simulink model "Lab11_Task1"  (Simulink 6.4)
settings: Solver=ode45  StartTime=0.0  StopTime=40  MaxStep=0.008  RelTol=1e-3
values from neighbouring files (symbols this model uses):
  B1 = 1/R1+D1    (= 5.99001338888)    [AGC_Data.m]
  D1 = 0.75/(2*pi*60)    (= 0.00198943678865)    [AGC_Data.m]
  DL1 = 1    [AGC_Data.m]
  DL2 = 0    [AGC_Data.m]
  K1 = 0.001*((2*pi*60))    (= 0.376991118431)    [AGC_Data.m]
  M1 = (2*H1)/(2*pi*60)    (= 0.0281173732796)    [AGC_Data.m]
  R1 = 0.167    [AGC_Data.m]
  T12 = 0.1    [AGC_Data.m]
  Tg1 = .26    (= 0.26)    [AGC_Data.m]
  thetar = 0    [AGC_Data.m]
  Ts1 = .26    (= 0.26)    [AGC_Data.m]

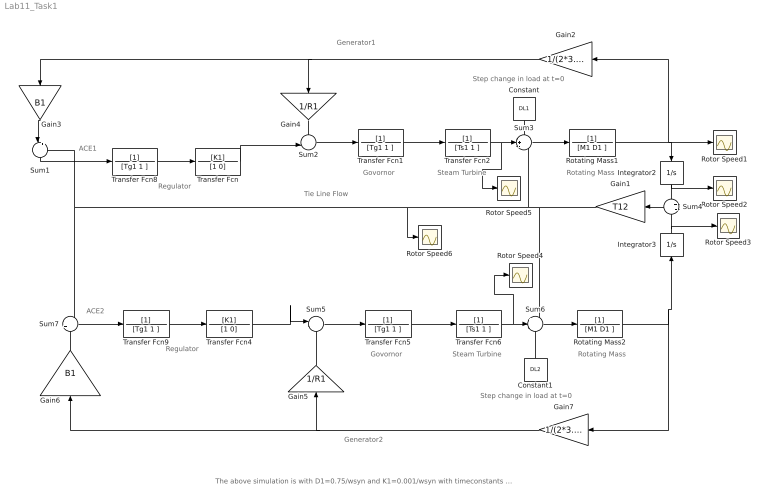
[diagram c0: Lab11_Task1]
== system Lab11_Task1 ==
  note: The above simulation is with D1=0.75/wsyn and K1=0.001/wsyn with timeconstants Tg1,Ts1 in seconds
  note: Generator1
  note: Generator2
  note: Rotating Mass
  note: Rotating Mass
  note: Step change in load at t=0
  note: Step change in load at t=0
  note: Tie Line Flow
  note: Govornor
  note: Steam Turbine
  note: Regulator
  note: Regulator
  note: Govornor
  note: Steam Turbine
  note: ACE1
  note: ACE2
  Constant : Constant  Orientation=down  Value=DL1  OutDataType=sfix(16)  ConRadixGroup=Use specified scaling  OutScaling=2^0  SampleTime=inf  FramePeriod=inf
  Constant1 : Constant  Orientation=up  Value=DL2  OutDataType=sfix(16)  ConRadixGroup=Use specified scaling  OutScaling=2^0  SampleTime=inf  FramePeriod=inf
  Gain1 : Gain  Orientation=left  Gain=T12
  Gain2 : Gain  Orientation=left  Gain=1/(2*3.14*60)
  Gain3 : Gain  Orientation=down  Gain=B1
  Gain4 : Gain  Orientation=down  Gain=1/R1
  Gain5 : Gain  Orientation=up  Gain=1/R1
  Gain6 : Gain  Orientation=up  Gain=B1
  Gain7 : Gain  Orientation=left  Gain=1/(2*3.14*60)
  Integrator2 : Integrator  Orientation=down  InitialCondition=thetar
  Integrator3 : Integrator  Orientation=up  InitialCondition=thetar
  Rotating Mass1 : TransferFcn  Denominator=[M1 D1 ]
  Rotating Mass2 : TransferFcn  Denominator=[M1 D1 ]
  Rotor Speed{1..6} (6 alike) : Scope
  Sum1 : Sum  Orientation=down  Inputs=|++
  Sum2 : Sum  Inputs=--
  Sum3 : Sum  Inputs=-+-
  Sum4 : Sum  Orientation=left  Inputs=+-
  Sum5 : Sum  Inputs=--
  Sum6 : Sum  Inputs=++-
  Sum7 : Sum  Inputs=-+
  Transfer Fcn : TransferFcn  Numerator=[K1]  Denominator=[1 0]
  Transfer Fcn{1,5,8..9} (4 alike) : TransferFcn  Denominator=[Tg1 1 ]
  Transfer Fcn2 : TransferFcn  Denominator=[Ts1 1 ]
  Transfer Fcn4 : TransferFcn  Numerator=[K1]  Denominator=[1 0]
  Transfer Fcn6 : TransferFcn  Denominator=[Ts1 1 ]
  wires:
  Sum1/1 -> Transfer Fcn8/1
  Gain3/1 -> Sum1/1
  Transfer Fcn1/1 -> Transfer Fcn2/1
  Gain4/1 -> Sum2/1
  Transfer Fcn/1 -> Sum2/2
  Sum2/1 -> Transfer Fcn1/1
  Transfer Fcn2/1 -> Sum3/2, Rotor Speed5/1
  Constant/1 -> Sum3/1
  Sum3/1 -> Rotating Mass1/1
  Rotating Mass1/1 -> Rotor Speed1/1, Integrator2/1, Gain2/1
  Integrator2/1 -> Sum4/1, Rotor Speed2/1
  Integrator3/1 -> Sum4/2, Rotor Speed3/1
  Rotating Mass2/1 -> Integrator3/1, Gain7/1
  Constant1/1 -> Sum6/3
  Transfer Fcn6/1 -> Sum6/2, Rotor Speed4/1
  Sum6/1 -> Rotating Mass2/1
  Gain6/1 -> Sum7/2
  Sum7/1 -> Transfer Fcn9/1
  Transfer Fcn4/1 -> Sum5/1
  Gain5/1 -> Sum5/2
  Sum5/1 -> Transfer Fcn5/1
  Transfer Fcn5/1 -> Transfer Fcn6/1
  Sum4/1 -> Gain1/1
  Gain1/1 -> Sum6/1, Sum3/3, Sum1/2, Sum7/1, Rotor Speed6/1
  Transfer Fcn8/1 -> Transfer Fcn/1
  Transfer Fcn9/1 -> Transfer Fcn4/1
  Gain2/1 -> Gain3/1, Gain4/1
  Gain7/1 -> Gain6/1, Gain5/1
